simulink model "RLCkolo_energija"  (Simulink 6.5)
settings: Solver=ode45  StartTime=0.0  StopTime=2  RelTol=1e-6
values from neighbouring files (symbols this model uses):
  A = [-R/L -1/L; 1/C 0]    [primer_7_4c.m]
  C = str2num(C)    [patuvacki_bran_1.m]    (also in primer_7_3.m = 0.0001; primer_7_4.m = 0.0001; primer_7_4a.m = 0.0001; primer_7_4c.m = 0.0001)
undefined symbols (not defined in the file or in its folder): B, blocks, Continuous, D, powergui, x0, ZData
libraries: powerlib x5

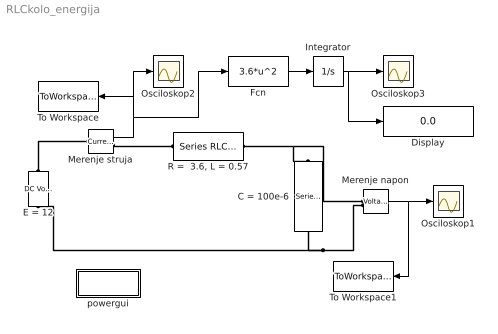
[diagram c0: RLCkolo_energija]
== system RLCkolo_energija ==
  C = 100e-6 : powerlib/Elements/Series RLC Branch  Orientation=down  DialogController=PMDialogs.PMDefaultMaskDlg  PhysicalDomain=powersysdomain  SubClassName=unknown  LeftPortType=p1  RightPortType=p1  LConnTagsString=__new0  RConnTagsString=__new0  BranchType=C  Resistance=1  Inductance=1e-3  SetiL0=off  InitialCurrent=0  Capacitance=100e-6  Setx0=on  InitialVoltage=0  Measurements=Branch voltage
  Display : Display
  E = 12 : powerlib/Electrical Sources/DC Voltage Source  Orientation=up  DialogController=PMDialogs.PMDefaultMaskDlg  SystemSampleTime=-1  Amplitude=12  Measurements=None
  Fcn : Fcn  Expr=3.6*u^2
  Integrator : Integrator
  Merenje napon : powerlib/Measurements/Voltage Measurement  DialogController=PMDialogs.PMDefaultMaskDlg  SystemSampleTime=-1  PhasorSimulation=off  OutputType=Complex  PSBequivalent=0
  Merenje struja : powerlib/Measurements/Current Measurement  DialogController=PMDialogs.PMDefaultMaskDlg  SystemSampleTime=-1  PhasorSimulation=off  OutputType=Complex  PSBequivalent=0
  Osciloskop1 : Scope
  Osciloskop2 : Scope
  Osciloskop3 : Scope
  "R =  3.6, L = 0.57" : powerlib/Elements/Series RLC Branch  DialogController=PMDialogs.PMDefaultMaskDlg  PhysicalDomain=powersysdomain  SubClassName=unknown  LeftPortType=p1  RightPortType=p1  LConnTagsString=__new0  RConnTagsString=__new0  BranchType=RL  Resistance=3.6  Inductance=0.57  SetiL0=on  InitialCurrent=0  Capacitance=100e-6  Setx0=on  InitialVoltage=0  Measurements=Branch current
  To Workspace : ToWorkspace  VariableName=struja  SampleTime=-1  SaveFormat=Array
  To Workspace1 : ToWorkspace  VariableName=napon  SampleTime=-1  SaveFormat=Array
  powergui : Subsystem  AncestorBlock=powerlib/powergui  InitFcn=powergui( 'InitFcn_Callback' , gcb , 0 , [ ] );  mask(PSB option menu block){SimulationMode=Continuous, SampleTime=50e-6, echomessages=off, RestoreLinks=warning, x0status=blocks, Frange=[0:2:500], Ylog=off, Xlog=on, ShowGrid=off, save=off, variable=ZData, structure=, ZoomFFT=on, StartTime=0.0, cycles=1, DisplayStyle=1, fundamental=60, FreqAxis=off, MaxFrequency=1000, frequencyindice=0, frequencyindicesteady=1, RmsSteady=1, display=off, Ts=0, frequency=60, methode=off, HookPort=off, Interpol=off}
      mask prompts: SimulationMode "Simulation mode"; SampleTime "Sample time Ts (when simulation mode is Discrete) (s)"; echomessages "Echo  Messages"; RestoreLinks "Restore disabled links"; x0status "Initial electrical states status"; Frange "Impedance tool: Frequency Range"; Ylog "Impedance tool: Log impedance"; Xlog "Impedance tool: log Frequency"; ShowGrid "Impedance tool: grid"; save "Impedance tool: Save Data To Workspace"; variable "Impedance tool: Variable Name"; structure "Structure Name (PSBFFTSCOPE)"; ZoomFFT "ZoomFFT (PSBFFTSCOPE)"; StartTime "Start Time (PSBFFTSCOPE)"; cycles "Cycles (PSBFFTSCOPE)"; DisplayStyle "Display style (PSBFFTSCOPE)"; fundamental "Fundamental (PSBFFTSCOPE)"; FreqAxis "Frequency Axis (PSBFFTSCOPE)"; MaxFrequency "Max Frequency (PSBFFTSCOPE)"; frequencyindice "Load flow frequency (Hz)"; frequencyindicesteady "Frequency indice (STEADYSTATE)"; RmsSteady "RMS display (STEADYSTATE)"; display "Display Results"; Ts "OBSOLETE 1"; frequency "Phasor frequency (Hz)"; methode "Phasor simulation"; HookPort "Hook port"; Interpol "Interpolate"
      mask init:
      | powerlibroot = which('powersysdomain');
      | PSBroot = powerlibroot(1:end-16);
      | %
      | switch SimulationMode
      | 	case 1
      | 		message=sprintf('Continuous');
      | 	case 2
      |         SampleTimeeval=evalin('base',SampleTime,'NaN');
      |         if isnan(SampleTimeeval)
      |             message=sprintf('Warning !!,\nUndefined sample time');
      |         else
      |             message=sprintf('Discrete,\nTs = %.4g s.',SampleTimeeval);
      |         end
      | 	case 3
      | 		message=sprintf('Phasors');
      | end
      | if strcmp(bdroot,'powerlib')
      |   message='powergui';
      | end
      | power_initmask();
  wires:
  Merenje napon/1 -> Osciloskop1/1, To Workspace1/1
  Merenje struja/1 -> Osciloskop2/1, To Workspace/1, Fcn/1
  Fcn/1 -> Integrator/1
  Integrator/1 -> Osciloskop3/1, Display/1
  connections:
  "R =  3.6, L = 0.57"/RConn1 -- Merenje napon/LConn1 -- C = 100e-6/LConn1
  Merenje napon/LConn2 -- E = 12/LConn1 -- C = 100e-6/RConn1
  E = 12/RConn1 -- Merenje struja/LConn1
  Merenje struja/RConn1 -- "R =  3.6, L = 0.57"/LConn1

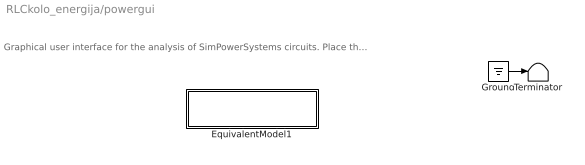
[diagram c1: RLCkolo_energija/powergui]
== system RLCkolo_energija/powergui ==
  note: Graphical user interface for the analysis of SimPowerSystems circuits. Place the Powergui block in the top-level of your model and double-click on it to open the GUI.
  EquivalentModel1 : Subsystem
  Ground : Ground
  Terminator : Terminator
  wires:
  Ground/1 -> Terminator/1

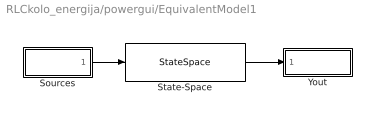
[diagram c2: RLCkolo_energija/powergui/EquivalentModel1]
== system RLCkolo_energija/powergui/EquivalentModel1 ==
  Sources : Subsystem
  State-Space : StateSpace  A=A  B=B  C=C  D=D  X0=x0
  Yout : Subsystem
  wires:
  Sources/1(u) -> State-Space/1
  State-Space/1 -> Yout/1(v,i)

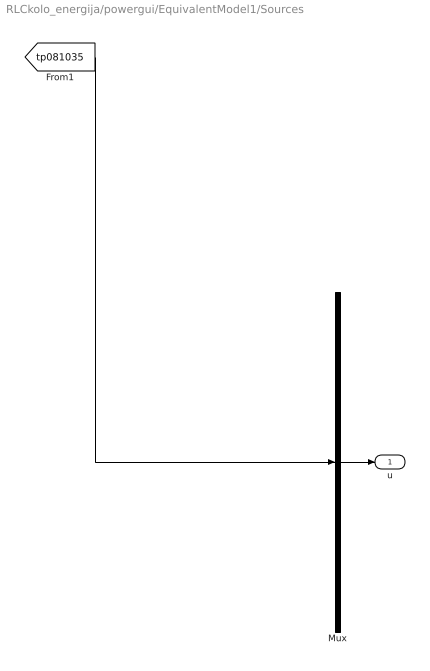
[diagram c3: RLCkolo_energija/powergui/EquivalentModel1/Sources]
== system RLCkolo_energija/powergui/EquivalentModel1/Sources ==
  Mux : Mux  Inputs=1
  u : Outport
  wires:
  Mux/1 -> u/1
  [tp081035] -> Mux/1

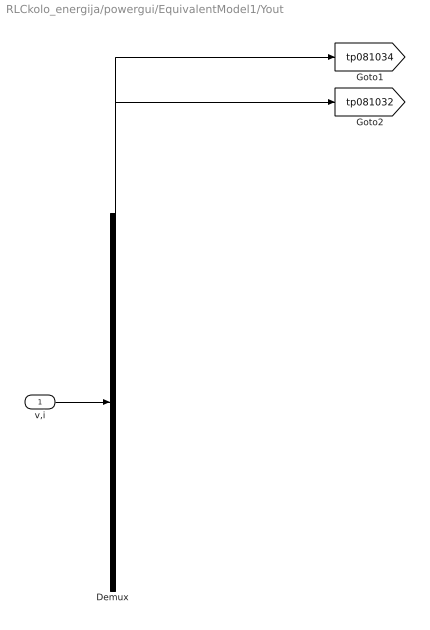
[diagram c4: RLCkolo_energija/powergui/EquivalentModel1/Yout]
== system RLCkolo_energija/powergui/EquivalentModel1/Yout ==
  v,i : Inport
  Demux : Demux  Outputs=[1 1]
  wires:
  v,i/1 -> Demux/1
  Demux/1 -> [tp081034]
  Demux/2 -> [tp081032]
